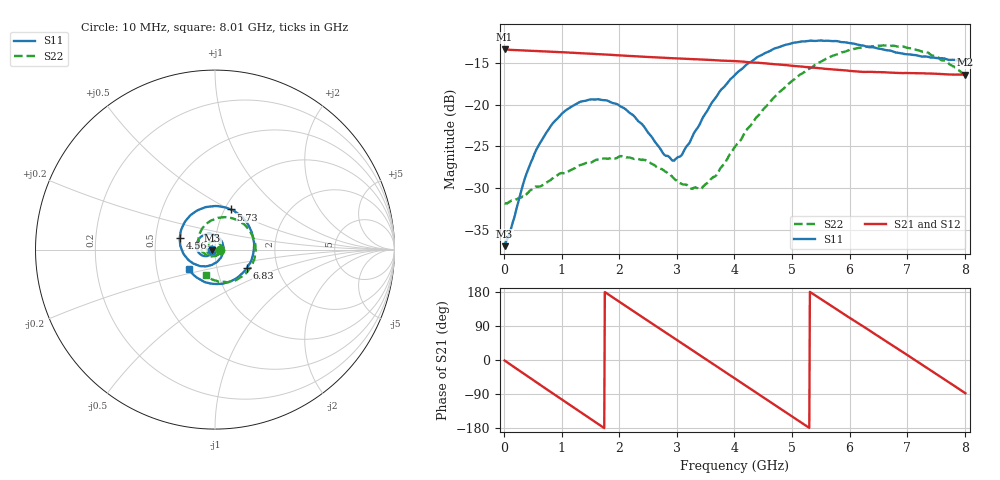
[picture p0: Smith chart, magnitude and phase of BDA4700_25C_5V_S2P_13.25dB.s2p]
!Agilent Technologies,E5071B,MY42404982,A.09.10
!Date: Mon Oct 20 13:32:47 2025
!Data & Calibration Information:
!Freq	S11:SOLT2(ON)	S21:SOLT2(ON)	S12:SOLT2(ON)	S22:SOLT2(ON)
# Hz S RI R 50
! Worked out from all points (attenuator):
!   801 points, 10 MHz to 8.01 GHz, reference 50 ohm
!   highest |S21| = -13.36 dB at 10 MHz (marker M1); lowest = -16.4 dB at 8 GHz (marker M2)
!   lowest |S11| = -36.9 dB at 10 MHz (marker M3), VSWR 1.03, Z = 48.6 - j0.147 ohm
!   |S11| at or under -10 dB: start of sweep to end of sweep
!   |S22| runs from -31.9 to -12.9 dB; largest |S21 - S12| = 0.0016
!   S11 on the Smith chart (normalised r, x): 10 MHz: 0.97, -0.00; 4.56 GHz: 0.67, +0.09; 5.73 GHz: 1.07, +0.51; 6.83 GHz: 1.40, -0.30; 8.01 GHz: 0.73, -0.16
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1e7  -0.0141 -0.00151  0.2148 -0.00479  0.2148 -0.00484  0.0257 -0.000983
3.8e8  -0.0261 -0.0272  0.162 -0.1357  0.1619 -0.1359  0.0208 -0.02
5.8e8  -0.0422 -0.0359  0.1028 -0.1828  0.1028 -0.1829  0.0131 -0.0296
8.8e8  -0.0731 -0.0321  -0.00577 -0.2074  -0.00578 -0.2075  -0.0097 -0.0356
1.35e9  -0.1037 0.0156  -0.1556 -0.1313  -0.1557 -0.1314  -0.0413 -0.0143
1.71e9  -0.0862 0.0629  -0.2001 -0.0118  -0.2002 -0.0116  -0.0443 0.0173
2.07e9  -0.0391 0.0877  -0.1649 0.1081  -0.1649 0.1083  -0.024 0.0425
2.68e9  0.0405 0.0394  0.0163 0.1915  0.0162 0.1914  0.026 0.0326
2.96e9  0.0453 -0.01  0.1034 0.1591  0.1035 0.159  0.0342 0.011
3.4e9  -0.00246 -0.0766  0.1823 0.0411  0.1826 0.041  0.0179 -0.0255
3.69e9  -0.0631 -0.0928  0.1771 -0.0525  0.1771 -0.053  -0.00975 -0.0368
4.01e9  -0.1349 -0.0678  0.12 -0.1376  0.1201 -0.1374  -0.0471 -0.0303
4.56e9  -0.196 0.0639  -0.0449 -0.1709  -0.0447 -0.1711  -0.0906 0.0387
4.98e9  -0.1458 0.1816  -0.1439 -0.0935  -0.1442 -0.0939  -0.0718 0.1168
5.35e9  -0.0407 0.2385  -0.1667 0.012  -0.167 0.0116  -0.00592 0.1676
5.73e9  0.0888 0.2236  -0.1211 0.1087  -0.121 0.1087  0.0894 0.1765
6.22e9  0.2023 0.1022  -0.000575 0.1575  0.001 0.1578  0.1975 0.0979
6.68e9  0.2043 -0.0554  0.1108 0.1097  0.1111 0.1097  0.2237 -0.0281
6.83e9  0.1784 -0.1013  0.1345 0.0775  0.1348 0.0769  0.2125 -0.0698
7.39e9  0.0206 -0.1916  0.1387 -0.0666  0.1386 -0.0669  0.1036 -0.1731
8e9  -0.1454 -0.1102  0.00839 -0.1512  0.00847 -0.1515  -0.0496 -0.1418
8.01e9  -0.1473 -0.1082  0.00571 -0.1514  0.00599 -0.1514  -0.0516 -0.14
